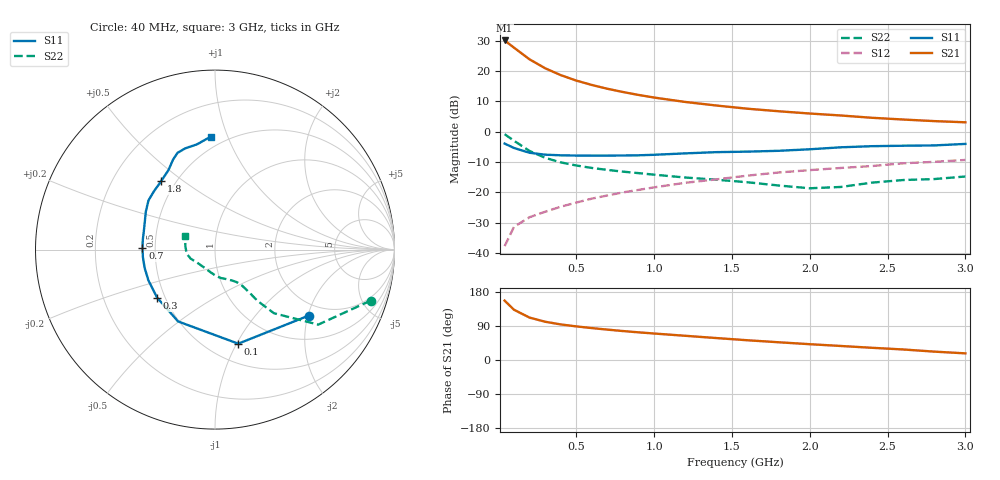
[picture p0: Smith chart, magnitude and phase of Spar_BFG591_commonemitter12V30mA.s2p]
! Filename:  BFG591C.S2P  Version:  4.0
! NXP part #: BFG591  Date: Jun 1994
! Bias condition: Vce=12V; Ic=30mA
#  MHz  S  MA  R  50
! Freq  S11  S21  S12  S22  !GUM [dB]
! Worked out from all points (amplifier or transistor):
!   21 points, 40 MHz to 3 GHz, reference 50 ohm
!   highest |S21| = 30.1 dB at 40 MHz (marker M1)
!   |S21| within 3 dB of that: start of sweep to 116.5 MHz
!   unconditionally stable (mu >= 1): 676.7 MHz to 2.195 GHz
!   at 300 MHz: K = 0.78, MSG = 23.7 dB, |S12| = -26.4 dB
!   at 1 GHz: K = 1.05, MAG = 13.4 dB, |S12| = -18.3 dB
!   at 3 GHz: K = 0.95, MSG = 6.2 dB, |S12| = -9.3 dB
!   S11 on the Smith chart (normalised r, x): 40 MHz: 1.63, -2.03; 100 MHz: 0.69, -1.02; 300 MHz: 0.45, -0.29; 700 MHz: 0.42, +0.01; 1.8 GHz: 0.42, +0.41; 3 GHz: 0.42, +0.87
40  0.639 -35.1  31.96 156.8  0.013 75.0  0.912 -18.2
100  0.54 -76.1  24.35 132.6  0.027 62.5  0.711 -36.0
200  0.45 -117.2  15.61 111.9  0.039 57.7  0.483 -47.2
300  0.419 -140.2  11.14 101.0  0.048 59.1  0.372 -50.3
400  0.409 -155.0  8.583 93.9  0.058 61.1  0.313 -51.2
500  0.405 -165.5  6.977 88.7  0.068 63.0  0.278 -52.1
600  0.404 -174.0  5.901 84.2  0.079 64.0  0.253 -53.0
700  0.404 179.0  5.111 80.2  0.089 65.0  0.235 -54.3
800  0.406 172.3  4.518 76.4  0.1 65.5  0.22 -56.0
900  0.409 166.0  4.042 73.0  0.11 66.0  0.208 -58.3
1000  0.417 160.3  3.661 69.9  0.121 65.9  0.196 -61.3
1200  0.44 151.1  3.098 63.9  0.144 65.2  0.176 -69.0
1400  0.461 143.5  2.706 57.9  0.164 63.9  0.162 -78.1
1600  0.47 136.6  2.396 52.1  0.189 63.3  0.147 -87.8
1800  0.485 128.3  2.177 46.8  0.213 60.5  0.13 -99.7
2000  0.514 120.2  1.996 41.7  0.233 59.1  0.117 -120.5
2200  0.554 114.9  1.853 37.0  0.253 57.1  0.123 -143.7
2400  0.578 111.2  1.698 32.2  0.272 56.3  0.145 -159.8
2600  0.588 106.4  1.59 27.8  0.302 52.9  0.16 -172.1
2800  0.595 99.7  1.497 22.1  0.319 49.0  0.166 173.5
3000  0.63 92.1  1.431 17.5  0.343 47.6  0.183 155.3
